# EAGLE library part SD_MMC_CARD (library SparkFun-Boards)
SD MMC Card Footprint Mechanical footprint with connectors of an SD/MMC card- NOT a socket! SparkFun Products: Electric Imp microSD Card with SD adapter
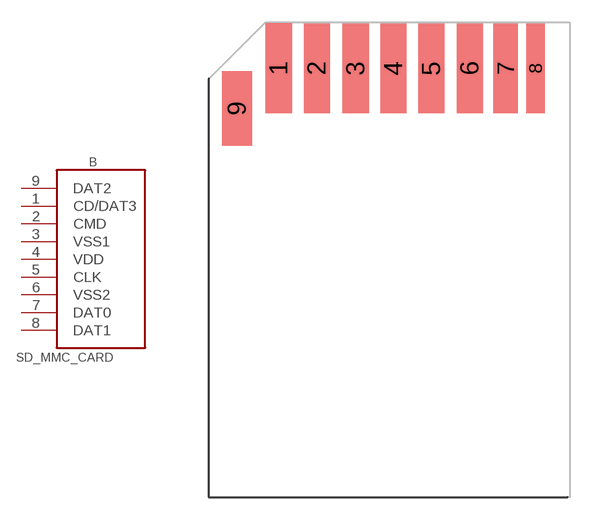
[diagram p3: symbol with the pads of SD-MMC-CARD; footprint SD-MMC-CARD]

Designator prefix B

## SD_MMC_CARDSD_PCB  [SD-MMC-CARD]
1  CD/DAT3
2  CMD
3  VSS1
4  VDD
5  CLK
6  VSS2
7  DAT0
8  DAT1
9  DAT2

## Footprint SD-MMC-CARD (pad centres in mm)
smd 1.75 x 6: 1 -6.745,14.713; 2 -4.195,14.703; 3 -1.6,14.703; 4 0.93,14.703; 5 3.465,14.703; 6 6.03,14.703
smd 1.65 x 6: 7 8.43,14.703
smd 1.25 x 6: 8 10.43,14.703
smd 2 x 5: 9 -9.53,12.03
